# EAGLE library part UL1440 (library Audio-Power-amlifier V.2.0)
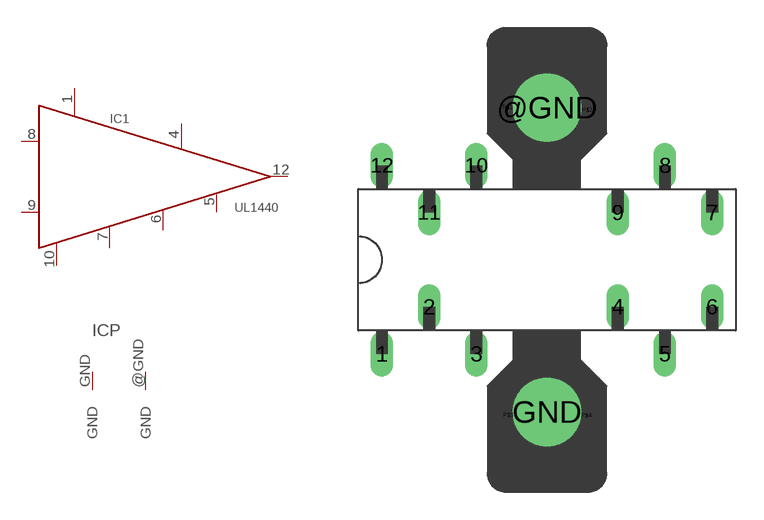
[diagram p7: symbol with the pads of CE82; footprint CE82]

Designator prefix IC; gates 1=UL1440 P=2GND

## UL1440T  [CE82]
1  1:VCC  pwr
4  1:BOSTRAP  pas
5  1:FCORE  pas
6  1:F_BACK  pas
7  1:TW  pas
8  1:IN  pas
9  1:GND  pwr
10  1:GND  pwr
12  1:OUT  pas
@GND  P:GND  pwr
GND  P:GND  pwr

## Footprint CE82 (pad centres in mm)
Package DIL 16 (CE83)
drill 0.7 long: 1 -8.89,-5.08; 2 -6.35,-2.54; 3 -3.81,-5.08; 4 3.81,-2.54; 5 6.35,-5.08; 6 8.89,-2.54; 7 8.89,2.54; 8 6.35,5.08; 9 3.81,2.54; 10 -3.81,5.08; 11 -6.35,2.54; 12 -8.89,5.08
drill 3.8: @GND 0,8.2; GND 0,-8.2
drill 0 pad 0.254: P$1 -2.12,8.22; P$2 2.17,8.07; P$3 -2.08,-8.37; P$4 2.12,-8.39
